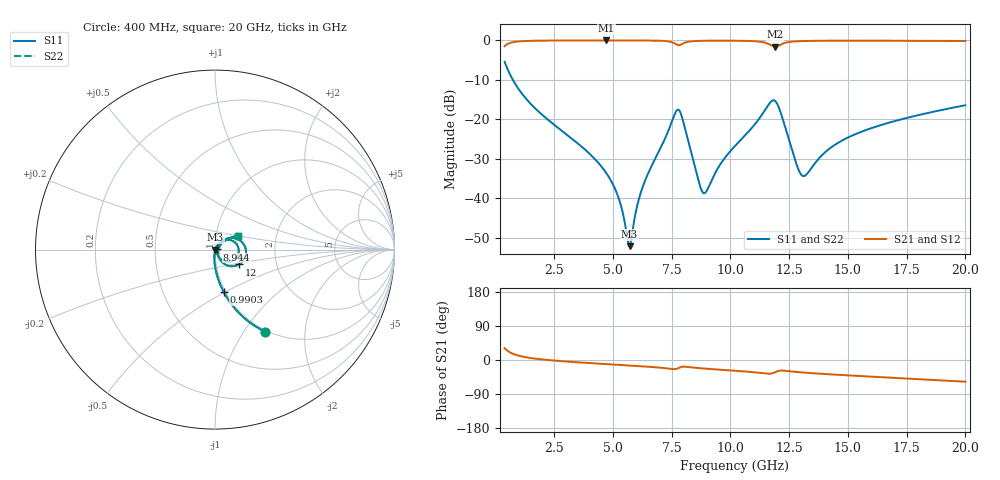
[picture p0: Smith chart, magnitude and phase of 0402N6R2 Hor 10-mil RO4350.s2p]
# GHz S MA R 50
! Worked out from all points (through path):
!   1960 points, 400 MHz to 20 GHz, reference 50 ohm
!   highest |S21| = -0.02 dB at 4.722 GHz (marker M1); lowest = -1.6 dB at 11.91 GHz (marker M2)
!   group delay of S21, straight-line fit = 9.03 ps
!   lowest |S11| = -52.1 dB at 5.713 GHz (marker M3), VSWR 1.00, Z = 50.2 - j0.0644 ohm
!   |S11| at or under -10 dB: 751.6 MHz to end of sweep
!   |S22| runs from -52.1 to -5.4 dB; largest |S21 - S12| = 0
!   S11 on the Smith chart (normalised r, x): 400 MHz: 0.98, -1.25; 990.3 MHz: 0.98, -0.50; 8.944 GHz: 1.02, +0.00; 12 GHz: 1.29, -0.22; 20 GHz: 1.28, +0.20
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0.4  0.5345 -58.7  0.8447 31.3  0.8447 31.3  0.5345 -58.7
0.9903012  0.243 -78.3  0.9692 11.5  0.9692 11.5  0.243 -78.3
3.671669  0.04528 -94.9  0.9973 -6.8  0.9973 -6.8  0.04528 -94.9
4.722205  0.02093 -95.8  0.9977 -10.8  0.9977 -10.8  0.02093 -95.8
5.252476  0.01003 -90.7  0.9976 -12.8  0.9976 -12.8  0.01003 -90.7
5.712711  0.002478 -15.0  0.9973 -14.5  0.9973 -14.5  0.002478 -15.0
6.202961  0.01207 57.7  0.9964 -16.4  0.9964 -16.4  0.01207 57.7
6.943338  0.03829 57.8  0.9907 -19.8  0.9907 -19.8  0.03829 57.8
7.543645  0.09883 33.1  0.9423 -23.9  0.9423 -23.9  0.09883 33.1
7.813783  0.1314 -13.8  0.8691 -20.7  0.8691 -20.7  0.1314 -13.8
8.704237  0.01454 -41.0  0.9859 -21.7  0.9859 -21.7  0.01454 -41.0
8.944359  0.01185 3.3  0.989 -22.9  0.989 -22.9  0.01185 3.3
10.205  0.04618 50.7  0.9897 -28.3  0.9897 -28.3  0.04618 50.7
11.46565  0.1298 28.8  0.9364 -35.5  0.9364 -35.5  0.1298 28.8
11.90587  0.1709 -18.9  0.8324 -32.1  0.8324 -32.1  0.1709 -18.9
11.99592  0.1568 -31.9  0.8428 -29.7  0.8428 -29.7  0.1568 -31.9
12.95641  0.02124 -33.2  0.9782 -32.3  0.9782 -32.3  0.02124 -33.2
13.16651  0.01929 -3.9  0.9826 -33.4  0.9826 -33.4  0.01929 -3.9
13.46667  0.02454 23.3  0.9862 -34.8  0.9862 -34.8  0.02454 23.3
14.63726  0.05155 42.2  0.9904 -39.3  0.9904 -39.3  0.05155 42.2
16.73834  0.09056 39.9  0.9894 -46.4  0.9894 -46.4  0.09056 39.9
20  0.1509 30.7  0.9823 -57.3  0.9823 -57.3  0.1509 30.7
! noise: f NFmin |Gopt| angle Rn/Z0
0.4  0.001184  0.7746  2.219  0.001072
2.571  0.004694  0.6573  6.984  0.002604
4.752  0.007782  0.6266  12.22  0.003861
6.933  0.01936  0.7642  17.51  0.01629
9.104  0.02386  0.7528  22.95  0.01872
11.29  0.05106  0.8506  28.24  0.06851
13.47  0.03368  0.7482  33.51  0.02472
15.64  0.02554  0.6433  38.27  0.01216
17.82  0.02539  0.6072  42.89  0.01046
20  0.02661  0.5913  47.35  0.01013
